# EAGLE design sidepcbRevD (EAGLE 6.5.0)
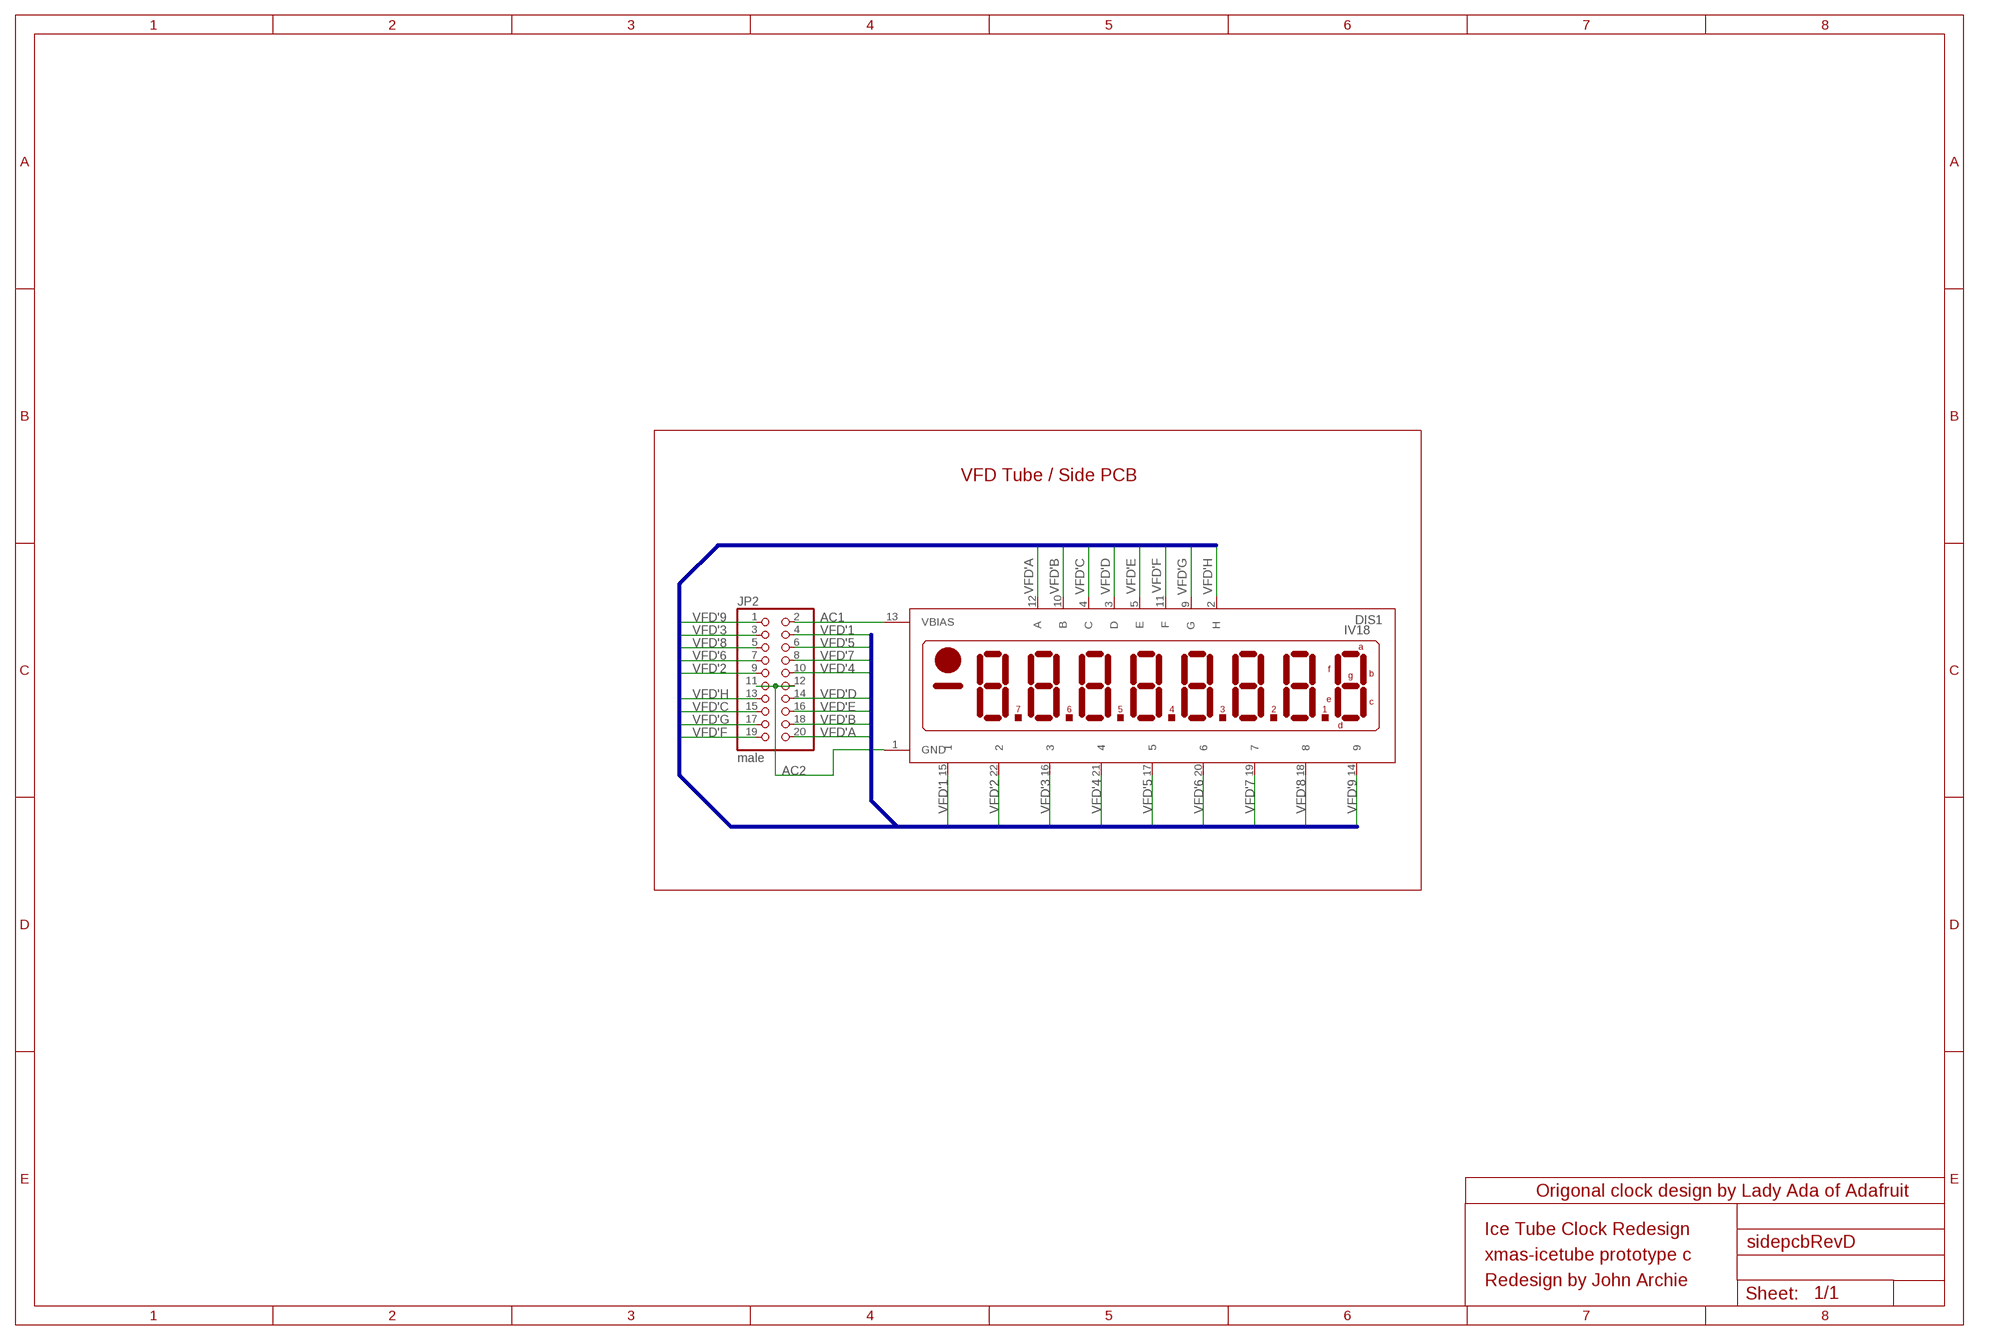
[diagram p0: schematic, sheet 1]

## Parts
DIS1  IV18  [IV18]
JP2  male  PINHD-2X10  [2X10]

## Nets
AC1: DIS1.13(VBIAS) JP2.2
AC2: DIS1.1(GND) JP2.11 JP2.12
VFD'1: DIS1.15 JP2.4
VFD'2: DIS1.22 JP2.9
VFD'3: DIS1.16 JP2.3
VFD'4: DIS1.21 JP2.10
VFD'5: DIS1.17 JP2.6
VFD'6: DIS1.20 JP2.7
VFD'7: DIS1.19 JP2.8
VFD'8: DIS1.18 JP2.5
VFD'9: DIS1.14 JP2.1
VFD'A: DIS1.12(A) JP2.20
VFD'B: DIS1.10(B) JP2.18
VFD'C: DIS1.4(C) JP2.15
VFD'D: DIS1.3(D) JP2.14
VFD'E: DIS1.5(E) JP2.16
VFD'F: DIS1.11(F) JP2.19
VFD'G: DIS1.9(G) JP2.17
VFD'H: DIS1.2(H) JP2.13

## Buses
VFD[1..9],VFD_A,VFD_B,VFD_C,VFD_D,VFD_E,VFD_F,VFD_G,VFD_H

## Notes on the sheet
- VFD Tube / Side PCB
- Origonal clock design by Lady Ada of Adafruit
- Ice Tube Clock Redesign
- xmas-icetube prototype c
- Redesign by John Archie

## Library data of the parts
DIS1 = vfd:IV18: LCD DISPLAY 8-character 7 segment
JP2 = pinhead:PINHD-2X10: PIN HEADER

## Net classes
0 default: clearance 0.205 mm

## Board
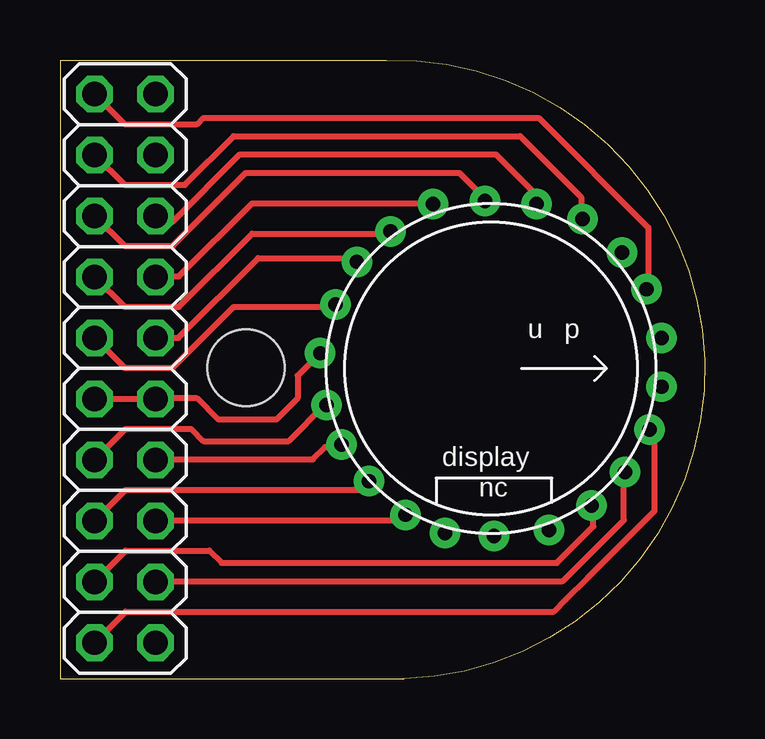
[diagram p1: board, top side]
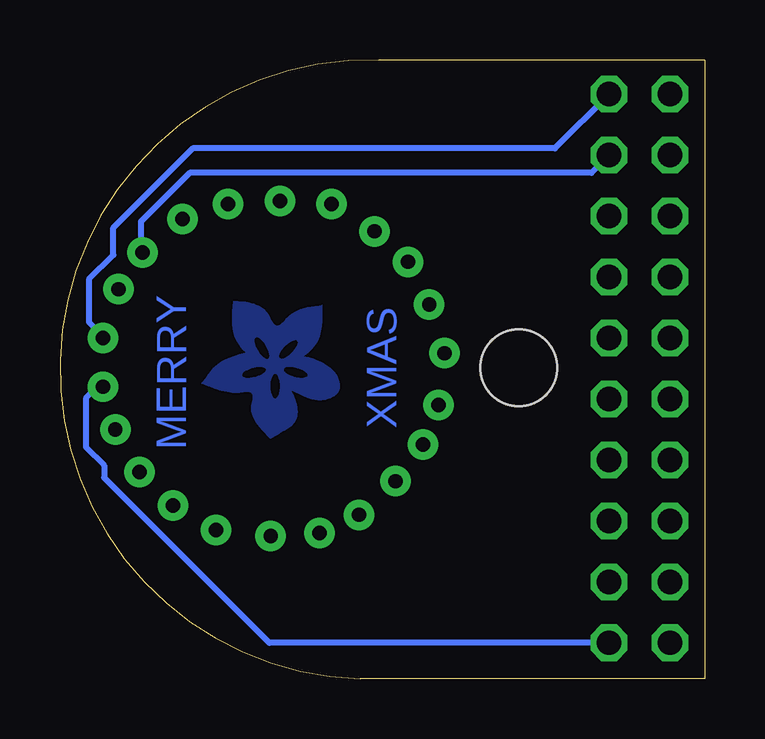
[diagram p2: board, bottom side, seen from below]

Size 26.86 x 25.78 mm. Coordinates in mm from the lower left corner, seen from the top.
Outline: 0,25.78 0,0 14.35,0 arc180 13.59,25.78 0,25.78
Copper layers (1*16): Top 0.0356mm / dielectric 1.5011mm / Bottom 0.0356mm
Design rules "LaenPCBOrder": minimum track width 6mil, minimum drill 13mil, track to track 6mil, track to pad 6mil, pad to pad 6mil, via to via 6mil, smd to smd 6mil, copper to edge 15mil, drill to drill 6mil, minimum pad ring 7mil, minimum via ring 7mil, stop-mask expansion 4mil, vias tented up to drill 0mil, thermal gap 10mil
Holes 3.2 mm at 7.75,12.95

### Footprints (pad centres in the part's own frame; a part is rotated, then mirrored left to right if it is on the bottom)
IV18 = drill 0.6 pad 1.27: 1 -0.635,-7.112; 2 1.524,-6.858; 3 3.175,-6.223; 4 4.699,-5.08; 5 6.096,-3.556; 6 6.858,-1.905; 7 6.985,0.127; 8 6.731,2.413; 9 5.715,4.191; 10 4.318,5.588; 11 2.54,6.604; 12 0.762,7.112; 13 -1.27,7.112; 14 -3.302,6.477; 15 -4.826,5.461; 16 -6.223,3.81; 17 -6.858,1.905; 18 -6.985,-0.254; 19 -6.858,-2.413; 20 -5.715,-4.191; 21 -4.445,-5.588; 22 -2.667,-6.477
2X10 = drill 1.016 octagon: 1 -11.43,-1.27; 2 -11.43,1.27; 3 -8.89,-1.27; 4 -8.89,1.27; 5 -6.35,-1.27; 6 -6.35,1.27; 7 -3.81,-1.27; 8 -3.81,1.27; 9 -1.27,-1.27; 10 -1.27,1.27; 11 1.27,-1.27; 12 1.27,1.27; 13 3.81,-1.27; 14 3.81,1.27; 15 6.35,-1.27; 16 6.35,1.27; 17 8.89,-1.27; 18 8.89,1.27; 19 11.43,-1.27; 20 11.43,1.27

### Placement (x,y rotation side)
DIS1  17.95,12.93 270 top
JP2  2.71,12.93 270 top

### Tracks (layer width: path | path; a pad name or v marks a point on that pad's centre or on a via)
AC1
  Bottom 0.254: JP2.2 6.25,22.1 21.34,22.1 24.64,18.8 24.64,17.65 25.65,16.64 25.65,14.86 25.07,14.27 DIS1.13 25.09,14.22
AC2
  Top 0.254: DIS1.1 9.91,12.63 9.91,11.68 9.02,10.79 6.6,10.79 5.72,11.68 4.01,11.68 JP2.12 JP2.11
N$6
  cutout Bottom: 17,14.08 16.97,14.05 16.96,14.01 16.97,13.96 17,13.88 17.05,13.78 17.16,13.64 17.24,13.56 17.34,13.48 17.45,13.4 17.54,13.36 17.62,13.34 17.67,13.35 17.7,13.37 17.71,13.39 17.72,13.42 17.72,13.47 17.71,13.51 17.67,13.58 17.62,13.69 17.52,13.8 17.45,13.87 17.34,13.96 17.27,14.02 17.19,14.06 17.11,14.09 17.06,14.1 17.02,14.1
N$7
  cutout Bottom: 18.17,13.37 18.16,13.4 18.15,13.46 18.16,13.53 18.18,13.63 18.24,13.77 18.29,13.86 18.36,13.98 18.43,14.06 18.49,14.13 18.56,14.18 18.61,14.2 18.65,14.22 18.69,14.21 18.72,14.18 18.74,14.14 18.75,14.11 18.75,14.07 18.74,14.02 18.73,13.98 18.69,13.86 18.66,13.79 18.61,13.68 18.56,13.6 18.51,13.53 18.42,13.43 18.37,13.39 18.31,13.35 18.26,13.33 18.23,13.32 18.2,13.34 18.18,13.35
N$8
  cutout Bottom: 18.29,12.87 18.29,12.9 18.3,12.92 18.33,12.94 18.37,12.96 18.43,12.98 18.49,12.98 18.53,12.98 18.61,12.98 18.68,12.97 18.77,12.95 18.86,12.93 18.96,12.9 19.04,12.86 19.11,12.83 19.18,12.78 19.22,12.74 19.25,12.69 19.26,12.65 19.25,12.61 19.22,12.58 19.17,12.56 19.12,12.55 19.08,12.54 18.95,12.54 18.85,12.56 18.76,12.57 18.69,12.59 18.62,12.62 18.54,12.65 18.46,12.69 18.4,12.73 18.37,12.75 18.33,12.78 18.31,12.81 18.3,12.84 18.29,12.86
N$11
  cutout Bottom: 18.08,12.19 18.07,12.06 18.06,11.94 18.02,11.83 17.99,11.76 17.96,11.71 17.91,11.68 17.88,11.69 17.85,11.7 17.81,11.74 17.78,11.8 17.75,11.86 17.74,11.91 17.73,11.97 17.72,12.04 17.71,12.1 17.71,12.3 17.72,12.38 17.73,12.44 17.74,12.48 17.76,12.53 17.78,12.58 17.8,12.61 17.81,12.64 17.84,12.66 17.86,12.68 17.88,12.69 17.91,12.69 17.94,12.68 17.97,12.64 17.99,12.61 18.02,12.57 18.03,12.52 18.05,12.45 18.07,12.36
N$13
  cutout Bottom: 16.79,12.54 16.72,12.55 16.66,12.56 16.62,12.57 16.59,12.59 16.57,12.61 16.56,12.63 16.56,12.66 16.57,12.69 16.58,12.72 16.61,12.76 16.66,12.8 16.75,12.85 16.85,12.89 16.91,12.92 16.99,12.94 17.05,12.96 17.15,12.97 17.22,12.98 17.27,12.98 17.32,12.98 17.38,12.98 17.43,12.97 17.48,12.95 17.51,12.93 17.52,12.92 17.53,12.89 17.53,12.86 17.51,12.82 17.48,12.78 17.44,12.75 17.4,12.72 17.35,12.69 17.3,12.66 17.26,12.64 17.2,12.62 17.11,12.59 17.01,12.57 16.94,12.55 16.87,12.54
N$14
  pour Bottom: 230 corners
VFD'1
  Bottom 0.254: JP2.4 4.72,21.08 21.46,21.08 23.49,19.05 23.49,17.84 DIS1.15
VFD'2
  Top 0.254: JP2.9 2.69,12.95 4.7,12.95 7.24,15.49 11.56,15.49 11.56,15.52 DIS1.22
VFD'3
  Top 0.254: JP2.3 2.69,20.57 5.21,20.57 7.24,22.61 19.18,22.61 21.72,20.07 21.72,19.3 21.76,19.26 DIS1.16
VFD'4
  Top 0.254: JP2.10 4.93,14.2 8.26,17.53 12.52,17.53 | 12.52,17.53 12.57,17.53 | 12.52,17.53 DIS1.21
VFD'5
  Top 0.254: DIS1.17 19.88,19.81 19.94,19.81 19.94,20.07 18.16,21.84 7.49,21.84 4.7,19.05 4.45,19.05 4.19,19.3 4.17,19.28 JP2.6
VFD'6
  Top 0.254: JP2.7 2.69,15.49 4.95,15.49 8,18.54 13.84,18.54 13.84,18.56 DIS1.20
VFD'7
  Top 0.254: DIS1.19 15.52,19.81 8,19.81 4.95,16.76 4.19,16.76 4.17,16.74 JP2.8
VFD'8
  Top 0.254: JP2.5 2.69,18.03 4.7,18.03 7.75,21.08 16.64,21.08 17.65,20.07 17.65,19.87 | 17.65,19.87 17.65,19.81 | 17.65,19.87 DIS1.18
VFD'9
  Top 0.254: JP2.1 2.69,23.11 5.72,23.11 5.97,23.37 19.94,23.37 24.51,18.8 24.51,16.26 24.46,16.26 DIS1.14
VFD'A
  Bottom 0.254: JP2.20 18.14,1.5 25.02,8.38 25.02,8.89 25.78,9.65 25.78,11.68 25.27,12.19 25.25,12.17 DIS1.12
VFD'B
  Top 0.254: JP2.18 4.01,4.06 20.95,4.06 23.49,6.6 23.49,8.64 23.52,8.64 DIS1.10
VFD'C
  Top 0.254: JP2.15 2.74,7.87 13.08,7.87 13.08,8.02 DIS1.4
VFD'D
  Top 0.254: JP2.14 4.01,9.14 10.54,9.14 11.05,9.65 11.63,9.65 DIS1.3
VFD'E
  Top 0.254: DIS1.5 14.17,6.6 4.01,6.6 JP2.16
VFD'F
  Top 0.254: JP2.19 2.74,2.79 20.57,2.79 21.08,3.3 21.97,4.19 24.77,6.99 24.77,10.18 DIS1.11
VFD'G
  Top 0.254: JP2.17 2.74,5.33 6.22,5.33 6.73,4.83 20.7,4.83 22.23,6.35 22.23,7.13 DIS1.9
VFD'H
  Top 0.254: JP2.13 2.74,10.41 5.46,10.41 5.97,9.91 9.53,9.91 11.05,11.43 11.07,11.43 DIS1.2

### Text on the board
Bottom: MERRY | XMAS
